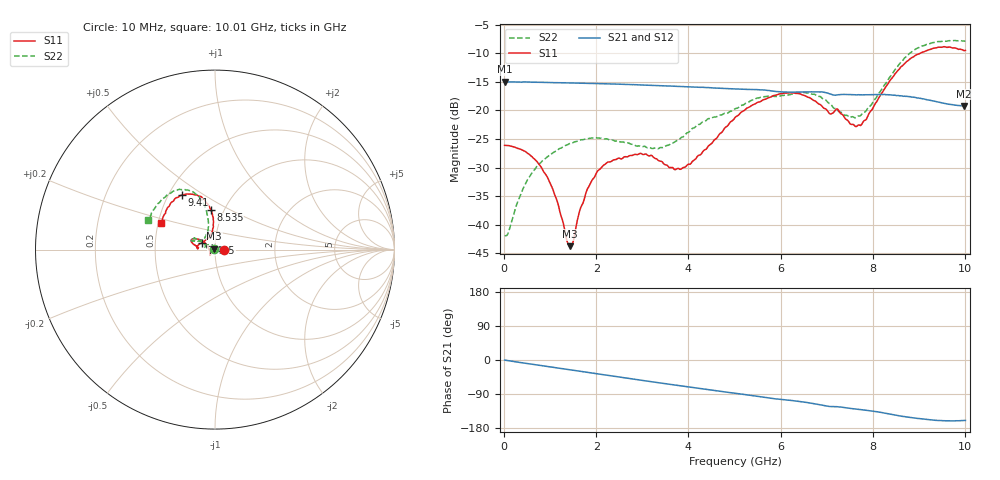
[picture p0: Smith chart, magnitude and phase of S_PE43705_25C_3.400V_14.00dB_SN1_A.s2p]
! Device ID: PE43705
! Serial: 1
! Insertion: A
! Impedance: 50 ohm
! Temp: 25C
! VDD: 3.400V
! Attenuation Step: 14.00dB
#  Hz  S  RI  R  50
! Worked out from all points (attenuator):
!   401 points, 10 MHz to 10.01 GHz, reference 50 ohm
!   highest |S21| = -14.97 dB at 10 MHz (marker M1); lowest = -19.2 dB at 9.985 GHz (marker M2)
!   lowest |S11| = -43.7 dB at 1.435 GHz (marker M3), VSWR 1.01, Z = 49.6 + j0.514 ohm
!   |S11| at or under -10 dB: start of sweep to 9.029 GHz
!   |S22| runs from -41.9 to -7.8 dB; largest |S21 - S12| = 0.0016
!   S11 on the Smith chart (normalised r, x): 10 MHz: 1.10, +0.00; 7.435 GHz: 0.86, +0.07; 8.535 GHz: 0.87, +0.40; 9.41 GHz: 0.58, +0.40; 10.01 GHz: 0.52, +0.17
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1e7  0.0496 0.000128  0.1785 -0.000729  0.1787 -0.000685  -0.00801 0.000565
4.6e8  0.0419 0.0127  0.1753 -0.0268  0.1753 -0.0264  -0.0115 0.0197
7.85e8  0.0283 0.0164  0.1706 -0.0442  0.1706 -0.0441  -0.0215 0.0271
1.085e9  0.0133 0.0134  0.1644 -0.0597  0.1644 -0.0597  -0.0329 0.0281
1.435e9  -0.00393 0.00518  0.1561 -0.0769  0.1561 -0.0767  -0.0451 0.025
1.685e9  -0.0144 -0.00324  0.1488 -0.0882  0.1489 -0.0881  -0.0515 0.0205
1.885e9  -0.0215 -0.00991  0.1424 -0.0969  0.1425 -0.0967  -0.0549 0.0164
2.21e9  -0.0264 -0.0221  0.131 -0.1098  0.131 -0.1098  -0.0557 0.00966
2.935e9  -0.0278 -0.0313  0.1012 -0.1333  0.1015 -0.1333  -0.0481 0.00885
3.36e9  -0.025 -0.0262  0.082 -0.1429  0.0822 -0.1427  -0.0451 0.0118
3.885e9  -0.0314 -0.00418  0.0576 -0.1508  0.0578 -0.1508  -0.0535 0.0243
5.01e9  -0.071 0.0497  0.00593 -0.154  0.00624 -0.1542  -0.0887 0.0531
5.985e9  -0.1267 0.0593  -0.0344 -0.1416  -0.0338 -0.1415  -0.119 0.0607
6.685e9  -0.121 0.0306  -0.0603 -0.1322  -0.0602 -0.1321  -0.129 0.0509
7.435e9  -0.0732 0.0389  -0.0818 -0.1109  -0.0817 -0.1113  -0.0714 0.0559
7.785e9  -0.0317 0.0721  -0.0909 -0.1024  -0.0905 -0.1027  -0.0492 0.0815
8.36e9  -0.0101 0.1787  -0.1086 -0.0836  -0.108 -0.0838  -0.0418 0.1891
8.535e9  -0.0245 0.2199  -0.1125 -0.0748  -0.1115 -0.076  -0.0556 0.234
8.935e9  -0.0767 0.2951  -0.1162 -0.0576  -0.1158 -0.0568  -0.1243 0.3223
9.41e9  -0.1864 0.3035  -0.1113 -0.0412  -0.1111 -0.0417  -0.2324 0.3259
9.985e9  -0.2939 0.1564  -0.1026 -0.0383  -0.1026 -0.0385  -0.3628 0.1768
1.001e10  -0.3008 0.1476  -0.1027 -0.0386  -0.1032 -0.0393  -0.3707 0.1654
